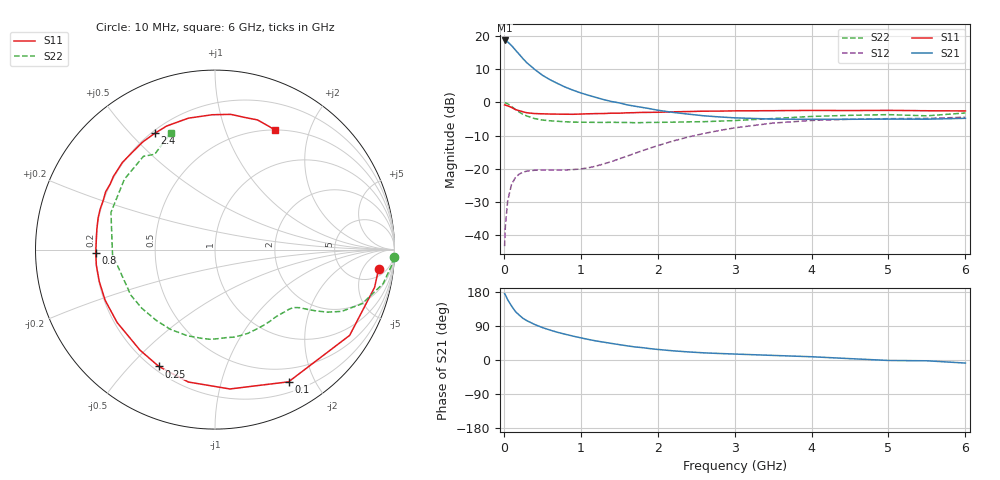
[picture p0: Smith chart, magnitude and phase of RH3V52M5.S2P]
! SIEMENS Small Signal Semiconductors
! BFR106
! Si NPN RF Bipolar Junction Transistor in SOT23
! VCE = 3.5 V  IC = 2.5 mA
! Common Emitter S-Parameters:  August  1996
# GHz  S  MA  R  50
!  f  S11  S21  S12  S22
! GHz  MAG  ANG  MAG  ANG  MAG  ANG  MAG  ANG
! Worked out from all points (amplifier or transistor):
!   36 points, 10 MHz to 6 GHz, reference 50 ohm
!   highest |S21| = 18.8 dB at 10 MHz (marker M1)
!   |S21| within 3 dB of that: start of sweep to 154.5 MHz
!   unconditionally stable (mu >= 1): 747.9 MHz to 2.003 GHz; 3.991 GHz to end of sweep
!   at 250 MHz: K = 0.35, MSG = 17.2 dB, |S12| = -21.1 dB
!   at 1.4 GHz: K = 1.23, MAG = 6.2 dB, |S12| = -17.9 dB
!   at 6 GHz: K = 1.02, MAG = -1.1 dB, |S12| = -4.5 dB
!   S11 on the Smith chart (normalised r, x): 10 MHz: 8, -11; 100 MHz: 0.32, -1.65; 250 MHz: 0.22, -0.61; 800 MHz: 0.20, -0.01; 2.4 GHz: 0.21, +0.59; 6 GHz: 0.50, +1.50
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0.01  0.9181 -6.7  8.681 175.1  0.0067 88.5  0.996 -2.4
0.02  0.9137 -13.3  8.646 171.7  0.0134 83.4  0.9902 -4.8
0.05  0.8895 -32.5  8.231 159.0  0.0325 72.3  0.9562 -11.4
0.1  0.843 -60.9  7.278 142.6  0.0577 58.6  0.8733 -20.2
0.15  0.7809 -83.9  6.23 128.1  0.073 47.9  0.7854 -26.0
0.2  0.7525 -101.4  5.359 118.4  0.0826 41.3  0.7165 -29.1
0.25  0.7223 -115.7  4.584 109.8  0.0882 35.9  0.6596 -31.2
0.3  0.6989 -126.7  3.99 103.7  0.0916 33.0  0.6239 -32.5
0.4  0.68 -143.3  3.17 93.8  0.0943 29.3  0.5712 -34.5
0.5  0.6741 -155.3  2.59 85.7  0.0953 28.3  0.5426 -36.5
0.6  0.6687 -164.7  2.211 79.0  0.0949 29.0  0.5286 -39.1
0.8  0.6643 -178.5  1.706 67.9  0.0953 34.0  0.5104 -45.2
1.1  0.6749 164.6  1.286 54.2  0.103 47.5  0.5016 -56.3
1.6  0.6978 144.2  0.922 37.4  0.1542 64.1  0.4988 -77.8
2.2  0.7225 123.7  0.708 24.2  0.2614 64.0  0.504 -107.7
2.4  0.7294 117.4  0.666 21.3  0.3009 61.0  0.509 -119.2
3  0.7471 101.4  0.586 15.7  0.4133 48.8  0.5332 -151.6
3.5  0.7515 91.2  0.56 12.1  0.488 37.4  0.5717 -177.2
4.5  0.7548 77.2  0.557 3.6  0.5575 16.3  0.6391 142.2
5  0.7603 71.9  0.561 -1.2  0.5691 8.1  0.6551 127.5
5.5  0.7501 66.7  0.559 -2.1  0.5744 4.2  0.6284 122.3
6  0.7453 63.4  0.576 -8.1  0.5988 -3.7  0.6942 110.9
